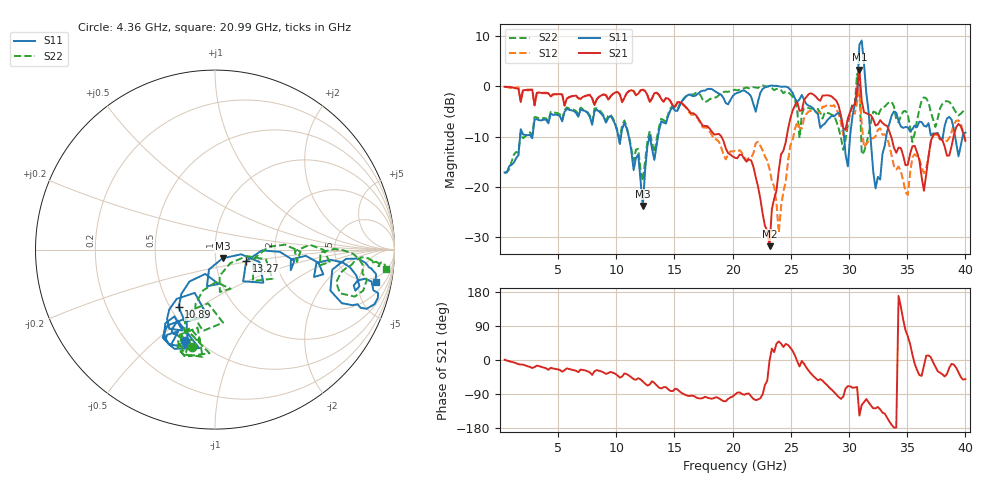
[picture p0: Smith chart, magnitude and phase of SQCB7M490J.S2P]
! Network Analyzer HP8722ES.07.66: Jul 25, 2000 Serial No. US39175408
! 27 Oct 2004  11:04:41
! Frequency  S11  S21  S12  S22
# HZ  S  DB R  50
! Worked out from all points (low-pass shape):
!   201 points, 400 MHz to 40 GHz, reference 50 ohm
!   highest |S21| = 3.36 dB at 30.89 GHz (marker M1); lowest = -31.9 dB at 23.17 GHz (marker M2)
!   |S21| within 3 dB of the highest: 30.74 GHz to 30.99 GHz (244.9 MHz wide, 0.794 % of centre)
!   lowest |S11| = -23.8 dB at 12.28 GHz (marker M3), VSWR 1.14, Z = 54.2 - j5.25 ohm
!   |S11| at or under -10 dB: start of sweep to 1.73 GHz; 11.07 GHz to 12.85 GHz (1.777 GHz wide, 14.9 % of centre); 31.84 GHz to 33.2 GHz (1.356 GHz wide, 4.17 % of centre)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
!   |S22| runs from -18.9 to 2.5 dB; largest |S21 - S12| = 0.66
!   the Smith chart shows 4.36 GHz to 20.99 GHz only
!   S11 on the Smith chart (normalised r, x): 4.36 GHz: 0.44, -0.63; 10.89 GHz: 0.55, -0.41; 13.27 GHz: 1.41, -0.18; 20.99 GHz: 3.75, -8.22
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4e8  -17.15 -92.4  -0.07 0.7  0.00 1.6  -17.37 -88.5
4.36e9  -5.41 -108.2  -2.00 -20.7  -2.01 -19.7  -5.09 -103.3
7.132e9  -4.78 -119.0  -2.09 -26.4  -2.16 -27.2  -4.57 -109.3
1.0894e10  -8.44 -122.3  -1.33 -37.3  -1.37 -37.8  -8.07 -106.8
1.228e10  -23.85 -48.7  -0.64 -56.9  -0.67 -57.6  -18.88 -41.2
1.327e10  -14.65 -20.0  -1.35 -60.3  -1.36 -61.2  -13.14 -13.8
1.3666e10  -8.83 -2.0  -1.63 -72.9  -1.72 -73.7  -8.17 4.1
2.02e10  -1.48 -5.1  -14.24 -91.1  -12.90 -78.6  -0.66 -5.6
2.0992e10  -0.79 -11.5  -14.41 -91.8  -14.13 -78.6  -0.37 -6.4
2.317e10  0.12 -3.5  -31.86 -1.2  -16.48 -93.2  0.07 -26.2
2.3962e10  0.02 -12.6  -16.70 48.8  -29.27 -48.9  -0.50 -43.6
2.4952e10  -0.64 -21.6  -6.44 32.5  -11.82 27.0  -1.54 -88.9
2.6932e10  -4.45 -23.0  -1.61 -42.4  -4.92 -40.4  -4.42 125.4
2.911e10  -5.26 -23.2  -3.88 -97.7  -5.41 -95.1  -8.37 25.4
3.01e10  -9.66 101.4  -5.04 -69.5  -5.52 -78.4  -5.19 -171.4
3.0694e10  -1.75 52.3  -0.59 -71.3  -3.14 -86.0  2.52 175.7
3.0892e10  8.33 -0.6  3.36 -146.7  0.01 -168.6  0.29 80.4
3.109e10  9.17 -62.5  -2.92 -118.5  -7.58 -133.2  -13.57 -170.1
3.1288e10  4.42 -80.8  -5.15 -111.3  -12.14 -117.1  -13.02 -148.4
3.1882e10  -11.19 -111.7  -5.74 -120.1  -10.34 -98.5  -7.16 166.5
3.3466e10  -7.37 -5.5  -8.98 -162.3  -11.78 -150.7  -3.11 138.9
4e10  -9.20 136.3  -10.88 -50.5  -10.73 -44.4  -4.50 -159.7
